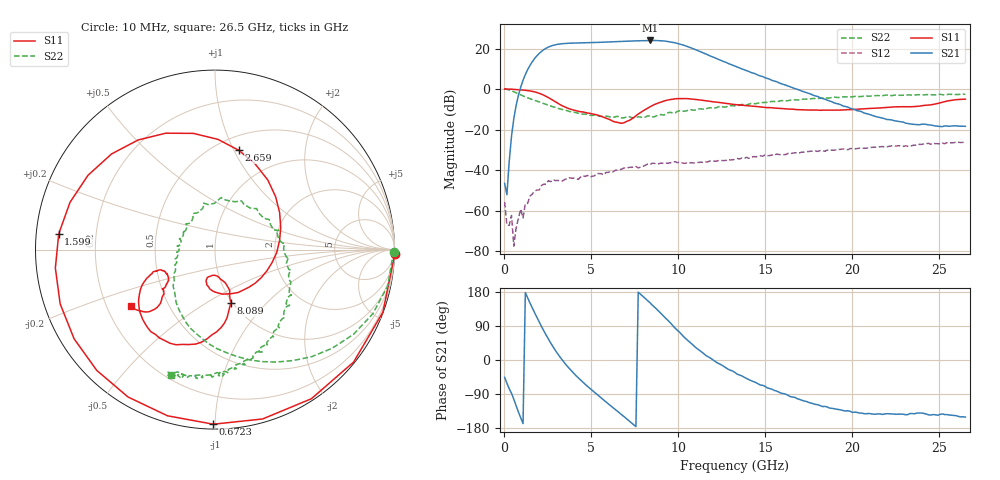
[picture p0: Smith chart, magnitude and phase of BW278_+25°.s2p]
!Agilent Technologies,N5242A,MY52422126,A.09.90.01
!Agilent N5242A: A.09.90.01
!Date: Wednesday, January 01, 2014 06:12:02
!Correction: S11(Full 2 Port with power(1,2))
!S21(Full 2 Port with power(1,2))
!S12(Full 2 Port with power(1,2))
!S22(Full 2 Port with power(1,2))
!S2P File: Measurements: S11, S21, S12, S22:
# Hz S  dB  R 50
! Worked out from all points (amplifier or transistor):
!   201 points, 10 MHz to 26.5 GHz, reference 50 ohm
!   highest |S21| = 24.0 dB at 8.354 GHz (marker M1)
!   |S21| within 3 dB of that: 2.6 GHz to 10.52 GHz (7.924 GHz wide, 121 % of centre)
!   unconditionally stable (mu >= 1): 141.4 MHz to end of sweep
!   at 4.381 GHz: K = 4.77, MAG = 23.3 dB, |S12| = -43.4 dB
!   at 13.26 GHz: K = 5.39, MAG = 12.7 dB, |S12| = -34.7 dB
!   at 26.5 GHz: K = 26.17, MAG = -13.3 dB, |S12| = -26.2 dB
!   S11 on the Smith chart (normalised r, x): 10 MHz: -4, -74; 672.2 MHz: 0.03, -0.99; 1.599 GHz: 0.07, +0.05; 2.659 GHz: 0.64, +1.05; 8.089 GHz: 0.98, -0.65; 26.5 GHz: 0.30, -0.28
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1e7  0.01 -1.5  -46.59 -45.7  -55.73 58.0  -0.04 -0.7
6.7225e8  -0.24 -90.6  -8.13 -120.8  -68.58 -166.2  -1.90 -47.9
1.20205e9  -0.64 -147.7  7.15 177.9  -56.53 -161.7  -3.88 -73.3
1.5994e9  -1.16 174.3  13.44 137.5  -51.89 167.2  -5.17 -89.0
2.26165e9  -3.05 112.9  19.42 77.1  -46.99 125.1  -7.17 -111.5
2.659e9  -4.90 76.5  21.18 44.9  -45.72 109.4  -8.37 -122.9
3.05635e9  -6.97 41.1  22.06 16.7  -45.12 97.3  -9.49 -131.5
3.4537e9  -8.79 8.1  22.46 -7.6  -44.71 84.9  -10.30 -139.7
4.5133e9  -11.32 -61.7  22.81 -58.6  -42.75 67.0  -12.43 -157.3
5.308e9  -12.76 -93.5  22.99 -90.6  -41.70 68.2  -13.03 -167.1
6.23515e9  -15.91 -105.2  23.33 -125.4  -40.94 62.3  -14.08 176.8
7.29475e9  -14.90 -75.6  23.70 -165.8  -38.64 48.8  -14.03 161.2
8.08945e9  -10.14 -73.5  23.93 162.7  -37.63 36.4  -13.90 140.1
8.35435e9  -8.87 -78.2  23.97 151.7  -37.40 35.9  -13.38 138.3
8.88415e9  -6.77 -88.9  23.87 128.3  -36.85 28.2  -12.70 122.3
9.67885e9  -5.07 -108.8  23.05 90.7  -36.06 19.1  -11.90 98.7
1.0606e10  -4.81 -130.8  20.71 49.0  -36.64 7.5  -10.34 62.8
1.16656e10  -5.87 -146.8  16.98 9.5  -36.05 4.5  -9.58 31.0
1.3255e10  -7.68 -157.2  11.27 -33.0  -34.74 -5.4  -8.36 1.1
1.77583e10  -10.36 -154.8  -3.11 -115.1  -30.62 -44.8  -4.66 -56.1
2.212915e10  -8.99 -143.0  -15.11 -141.9  -28.26 -84.9  -3.16 -85.7
2.65e10  -4.98 -146.2  -18.41 -150.6  -26.24 -134.0  -2.64 -109.4
